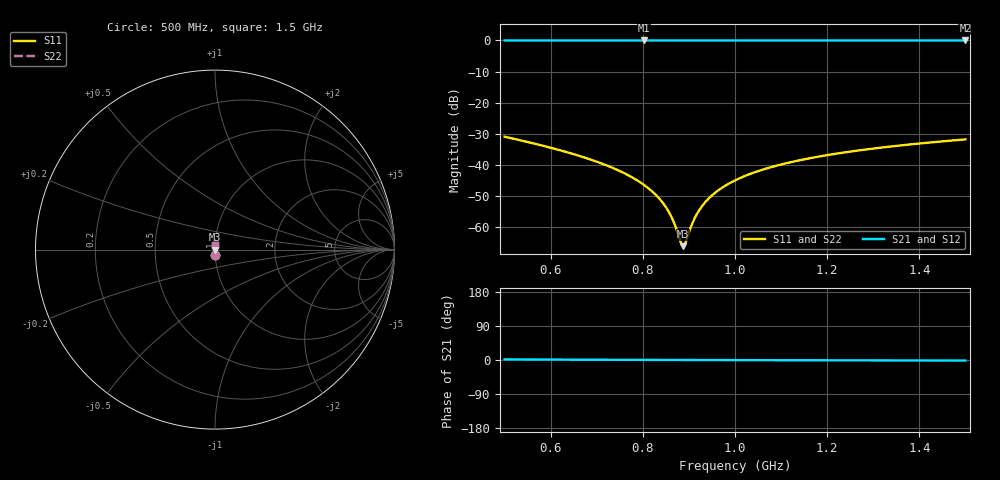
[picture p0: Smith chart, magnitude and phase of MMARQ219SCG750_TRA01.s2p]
! MMARQ219SCG750_TRA01  S-PARAMETER MODEL  ( General Type )
! Model Generated by TAIYO YUDEN Corporation (http://www.ty-top.com)
! Version 1.0
! TAIYO YUDEN Control No. 180601
! Copyright(c) 2018 TAIYO YUDEN CO.,LTD. All Rights Reserved.
! Product Description (link to TY-COMPAS)
! https://ds.yuden.co.jp/TYCOMPAS/or/detail?pn=MMARQ219SCG750JTRA01&u=M
! Products Name : Multilayer Ceramic Capacitors
! Characteristics :
!  Capacitance : 75 pF , Rated Voltage : 250V , TCC : CG / C0G
!  Case Size : 2.0 x 1.25 / 0.079 x 0.049 [mm/inch] , Thickness : 0.85 / 0.033 [mm/inch]
!  (Conditions: Temperature = 25 degC , DC Bias Current/Voltage = 0A / 0V)
! External Node Assignments :
!  1  o---| |---o  2
! GND o---------o GND
! Frequency Range : 500MHz  -  1500MHz  [ 401 STEP ]
# MHz S RI R 50
! Freq[MHz].  S11 Real  S11 Imag  S21 Real  S21 Imag  S12 Real  S12 Imag  S22 Real  S22 Imag
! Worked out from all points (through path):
!   401 points, 500 MHz to 1.5 GHz, reference 50 ohm
!   highest |S21| = 0.00 dB at 802.5 MHz (marker M1); lowest = 0.0 dB at 1.5 GHz (marker M2)
!   lowest |S11| = -66.2 dB at 887.5 MHz (marker M3), VSWR 1.00, Z = 50 - j0.000661 ohm
!   |S11| at or under -10 dB: start of sweep to end of sweep
!   |S22| runs from -66.2 to -31.0 dB; largest |S21 - S12| = 0
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500  0.0012 -0.0283  0.9988 0.0283  0.9988 0.0283  0.0012 -0.0283
590  0.000798 -0.0196  0.9992 0.0196  0.9992 0.0196  0.000798 -0.0196
667.5  0.000613 -0.0135  0.9994 0.0135  0.9994 0.0135  0.000613 -0.0135
745  0.000518 -0.00822  0.9995 0.00822  0.9995 0.00822  0.000518 -0.00822
775  0.000499 -0.00636  0.9995 0.00636  0.9995 0.00636  0.000499 -0.00636
802.5  0.000488 -0.00472  0.9995 0.00472  0.9995 0.00472  0.000488 -0.00472
835  0.000483 -0.00286  0.9995 0.00286  0.9995 0.00286  0.000483 -0.00286
847.5  0.000483 -0.00216  0.9995 0.00216  0.9995 0.00216  0.000483 -0.00216
860  0.000484 -0.00148  0.9995 0.00148  0.9995 0.00148  0.000484 -0.00148
870  0.000486 -0.000936  0.9995 0.000936  0.9995 0.000936  0.000486 -0.000936
882.5  0.000489 -0.00027  0.9995 0.00027  0.9995 0.00027  0.000489 -0.00027
887.5  0.00049 -6.6e-06  0.9995 6.6e-06  0.9995 6.6e-06  0.00049 -6.6e-06
892.5  0.000492 0.000256  0.9995 -0.000256  0.9995 -0.000256  0.000492 0.000256
905  0.000496 0.000905  0.9995 -0.000905  0.9995 -0.000905  0.000496 0.000905
915  0.000501 0.00142  0.9995 -0.00142  0.9995 -0.00142  0.000501 0.00142
932.5  0.000509 0.0023  0.9995 -0.0023  0.9995 -0.0023  0.000509 0.0023
962.5  0.000528 0.00378  0.9995 -0.00378  0.9995 -0.00378  0.000528 0.00378
1000  0.000556 0.00557  0.9994 -0.00557  0.9994 -0.00557  0.000556 0.00557
1070  0.000625 0.00877  0.9994 -0.00877  0.9994 -0.00877  0.000625 0.00877
1167.5  0.000749 0.0129  0.9993 -0.0129  0.9993 -0.0129  0.000749 0.0129
1335  0.00103 0.0195  0.999 -0.0195  0.999 -0.0195  0.00103 0.0195
1500  0.00136 0.0255  0.9986 -0.0255  0.9986 -0.0255  0.00136 0.0255
